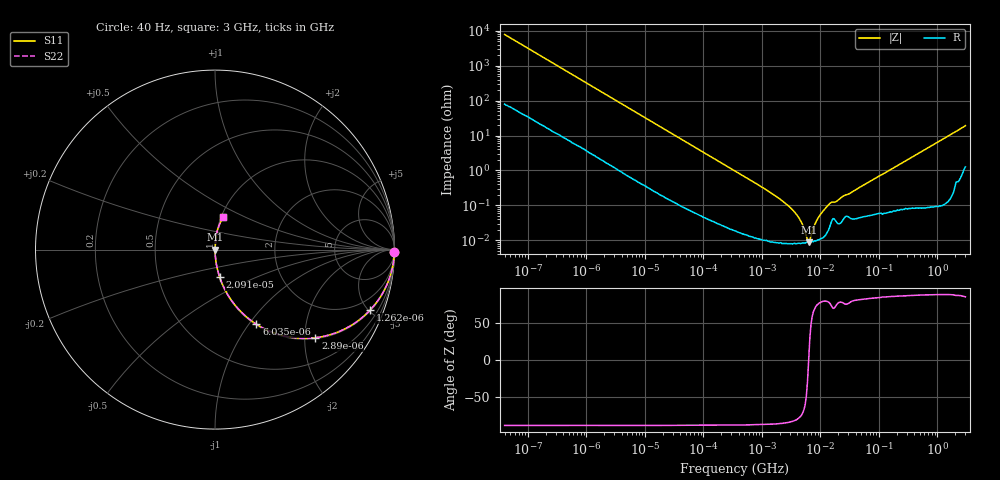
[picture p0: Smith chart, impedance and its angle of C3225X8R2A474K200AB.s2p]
! S-parameter Generated by TDK Corporation
! Copyright(C) 2015 TDK Corporation.
! All Rights Reserved.
! TDK P/N: C3225X8R2A474K200AB (Multilayer Ceramic Chip Capacitors)
! Property: C=470nF
! Size(LxWxT): 3.2x2.5x2mm, 0.126x0.098x0.079inches
! Model Type: s2p (Touchstone File Format Version 1.0)
! Frequency: DC=Yes Start=0.00004MHz Stop=3000MHz 396points Log-sweep
! Note: This model was converted from impedance.
! Model Generated on Jun. 23, 2015
! Hash(MD5):
! Port Assignments:
!  1 ---| |--- 2
! Applicable Conditions:
!  Temperature = 25 degC
!  DC Bias Voltage = 0 V
!  Small Signal Operation
! Terms and conditions regarding TDK Simulation Models
! (1)This simulation model is being provided solely for informational purposes. Please refer to the specifications of the products in terms of detailed characteristics of such products.
! (2)In no event shall TDK Corporation of any of its subsidiaries be liable for any loss or damage arising, directly or indirectly,
!  From any information contained in this simulation model, including, but not limited to loss or damages arising from any inaccuracies, omissions or errors in connection with such information.
! (3)Any and all copyrights on this simulation model are owned by TDK Corporation.
!  Duplication or redistribution of this simulation model without prior written permission from TDK Corporation is prohibited.
! (4)This simulation model is subject to any modification or change without any prior notice.
! (5)Neither TDK Corporation nor any of its subsidiaries shall make any warranty, express or implied,
!  Including but not limited to the correctness, implied warranties of merchantability and fitness for a particular purpose with respect to this simulation models.
! (6)The use of this simulation model shall be deemed to have consented to the terms and conditions hereof.
# MHz S MA R 50
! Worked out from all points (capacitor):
!   395 points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, 40 Hz to 3 GHz, reference 50 ohm
!   read as one part in series: C = 504 nF near 41.88 Hz
!   lowest |Z| = 8.85 mohm at 6.292 MHz (marker M1)
!   series resonance near 6.299 MHz, so ESL is about 1.3 nH
!   S11 on the Smith chart (normalised r, x): 40 Hz: open; 1.262 kHz: 1.06, -5.14; 2.89 kHz: 1.02, -2.26; 6.035 kHz: 1.01, -1.09; 20.91 kHz: 1.00, -0.32; 3 GHz: 1.03, +0.38
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4e-05  0.9998 -0.7  0.01269 88.7  0.01269 88.7  0.9998 -0.7
0.0002520917  0.9961 -4.5  0.07841 84.9  0.07841 84.9  0.9961 -4.5
0.000834128  0.9656 -14.4  0.2493 74.9  0.2493 74.9  0.9656 -14.4
0.001262176  0.9284 -21.2  0.3615 68.2  0.3615 68.2  0.9284 -21.2
0.002889976  0.7445 -41.3  0.6595 48.1  0.6595 48.1  0.7445 -41.3
0.006035228  0.4753 -61.0  0.8747 28.4  0.8747 28.4  0.4753 -61.0
0.01739424  0.1863 -78.6  0.9805 10.7  0.9805 10.7  0.1863 -78.6
0.02091006  0.1561 -80.4  0.986 9.0  0.986 9.0  0.1561 -80.4
0.3464102  0.009742 -88.4  0.9998 0.6  0.9998 0.6  0.009742 -88.4
3.013016  0.0008829 -84.8  0.9999 0.1  0.9999 0.1  0.0008829 -84.8
4.354128  0.0004211 -78.7  0.9999 0.0  0.9999 0.0  0.0004211 -78.7
5.234209  0.0002204 -67.6  0.9999 0.0  0.9999 0.0  0.0002204 -67.6
6.009156  0.0001019 -29.5  0.9999 0.0  0.9999 0.0  0.0001019 -29.5
6.292177  8.853e-05 -0.8  0.9999 0.0  0.9999 0.0  8.853e-05 -0.8
6.588528  0.0001025 29.6  0.9999 -0.0  0.9999 -0.0  0.0001025 29.6
7.22376  0.0001782 58.9  0.9999 -0.0  0.9999 -0.0  0.0001782 58.9
9.092863  0.000432 76.3  0.9999 -0.0  0.9999 -0.0  0.000432 76.3
15.08561  0.0012 75.1  0.9997 -0.1  0.9997 -0.1  0.0012 75.1
18.13479  0.001262 73.3  0.9996 -0.1  0.9996 -0.1  0.001262 73.3
150.6385  0.01008 85.8  0.9993 -0.6  0.9993 -0.6  0.01008 85.8
906.6656  0.05824 85.8  0.9974 -3.3  0.9974 -3.3  0.05824 85.8
3000  0.1861 75.5  0.9703 -10.7  0.9703 -10.7  0.1861 75.5
